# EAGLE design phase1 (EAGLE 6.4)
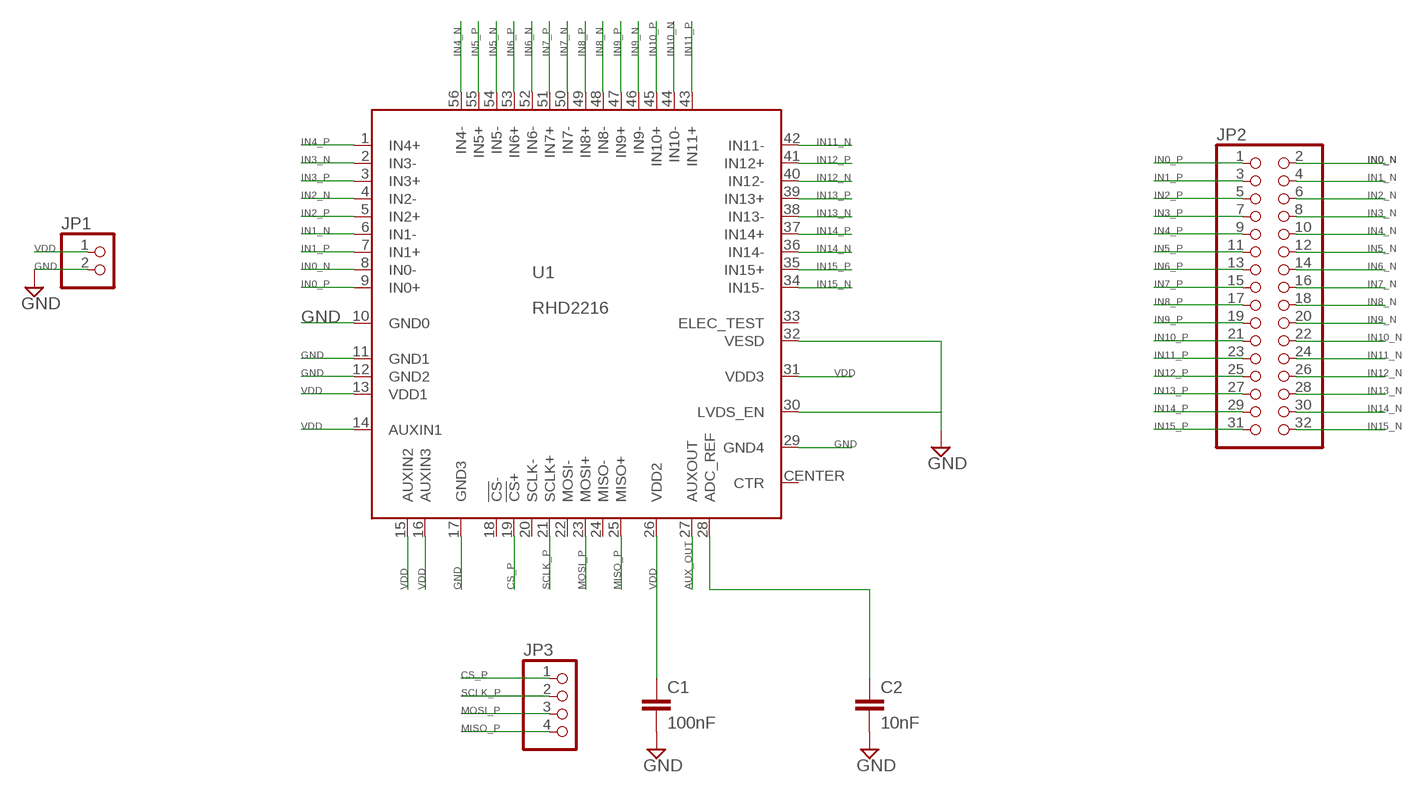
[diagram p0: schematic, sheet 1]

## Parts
C1  100nF  C2.5/2  [C2.5-2]
C2  10nF  C2.5/2  [C2.5-2]
JP1  PINHD-1X2  [1X02]
JP2  PINHD-2X16  [2X16]
JP3  PINHD-1X4  [1X04]
U1  RHD2216  [ZIF_QFN56_8_X_8_MLF00056A1]

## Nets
AUX_OUT: U1.27(AUXOUT)
CS_P: JP3.1 U1.19(!CS!+)
GND: C1.2 C2.2 JP1.2 U1.10(GND0) U1.11(GND1) U1.12(GND2) U1.17(GND3) U1.29(GND4) U1.30(LVDS_EN) U1.32(VESD)
IN0_N: JP2.2 U1.8(IN0-)
IN0_P: JP2.1 U1.9(IN0+)
IN1_N: JP2.4 U1.6(IN1-)
IN1_P: JP2.3 U1.7(IN1+)
IN2_N: JP2.6 U1.4(IN2-)
IN2_P: JP2.5 U1.5(IN2+)
IN3_N: JP2.8 U1.2(IN3-)
IN3_P: JP2.7 U1.3(IN3+)
IN4_N: JP2.10 U1.56(IN4-)
IN4_P: JP2.9 U1.1(IN4+)
IN5_N: JP2.12 U1.54(IN5-)
IN5_P: JP2.11 U1.55(IN5+)
IN6_N: JP2.14 U1.52(IN6-)
IN6_P: JP2.13 U1.53(IN6+)
IN7_N: JP2.16 U1.50(IN7-)
IN7_P: JP2.15 U1.51(IN7+)
IN8_N: JP2.18 U1.48(IN8-)
IN8_P: JP2.17 U1.49(IN8+)
IN9_N: JP2.20 U1.46(IN9-)
IN9_P: JP2.19 U1.47(IN9+)
IN10_N: JP2.22 U1.44(IN10-)
IN10_P: JP2.21 U1.45(IN10+)
IN11_N: JP2.24 U1.42(IN11-)
IN11_P: JP2.23 U1.43(IN11+)
IN12_N: JP2.26 U1.40(IN12-)
IN12_P: JP2.25 U1.41(IN12+)
IN13_N: JP2.28 U1.38(IN13-)
IN13_P: JP2.27 U1.39(IN13+)
IN14_N: JP2.30 U1.36(IN14-)
IN14_P: JP2.29 U1.37(IN14+)
IN15_N: JP2.32 U1.34(IN15-)
IN15_P: JP2.31 U1.35(IN15+)
MISO_P: JP3.4 U1.25(MISO+)
MOSI_P: JP3.3 U1.23(MOSI+)
N$1: C2.1 U1.28(ADC_REF)
SCLK_P: JP3.2 U1.21(SCLK+)
VDD: C1.1 JP1.1 U1.13(VDD1) U1.14(AUXIN1) U1.15(AUXIN2) U1.16(AUXIN3) U1.26(VDD2) U1.31(VDD3)
Unconnected: U1.18(!CS!-) U1.20(SCLK-) U1.22(MOSI-) U1.24(MISO-) U1.33(ELEC_TEST)

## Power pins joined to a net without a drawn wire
CTR: U1.CENTER(CTR)

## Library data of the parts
C1 C2 = capacitor-wima:C: CAPACITOR
JP1 = pinhead:PINHD-1X2: PIN HEADER
JP2 = pinhead:PINHD-2X16: PIN HEADER
JP3 = pinhead:PINHD-1X4: PIN HEADER
U1 = RHD2000:RHD2216

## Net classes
0 default: clearance 0.355 mm

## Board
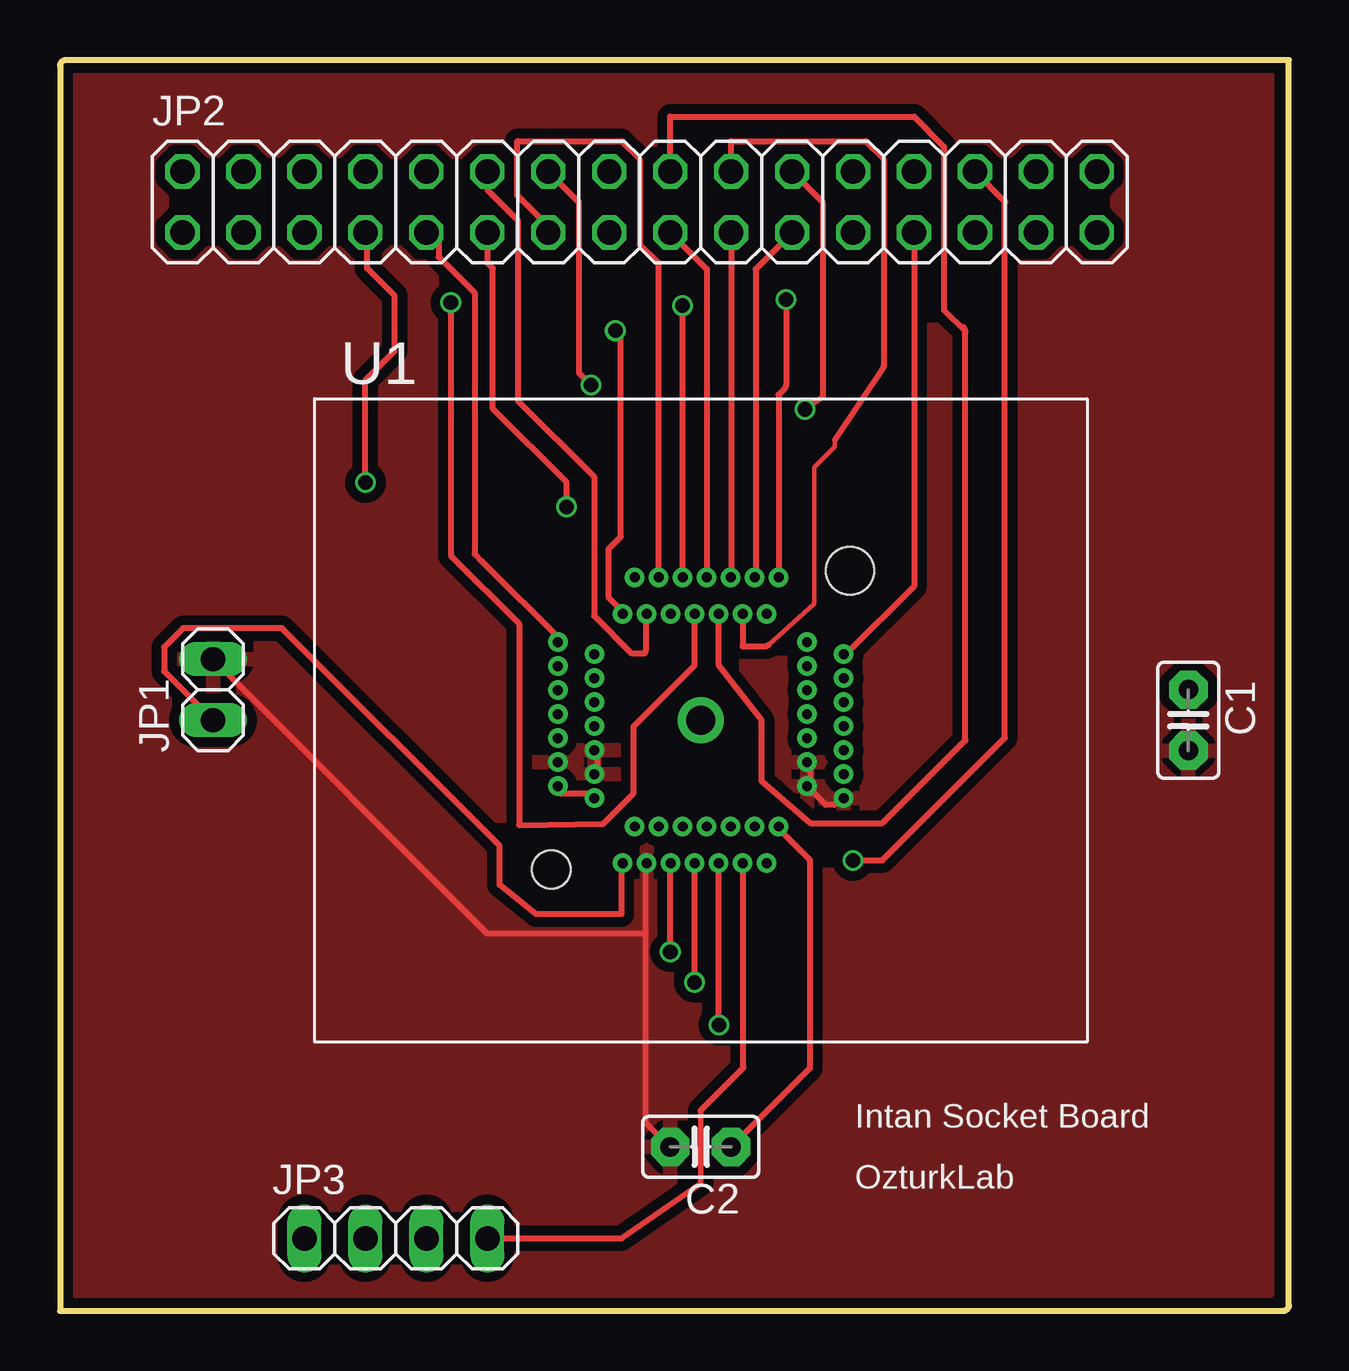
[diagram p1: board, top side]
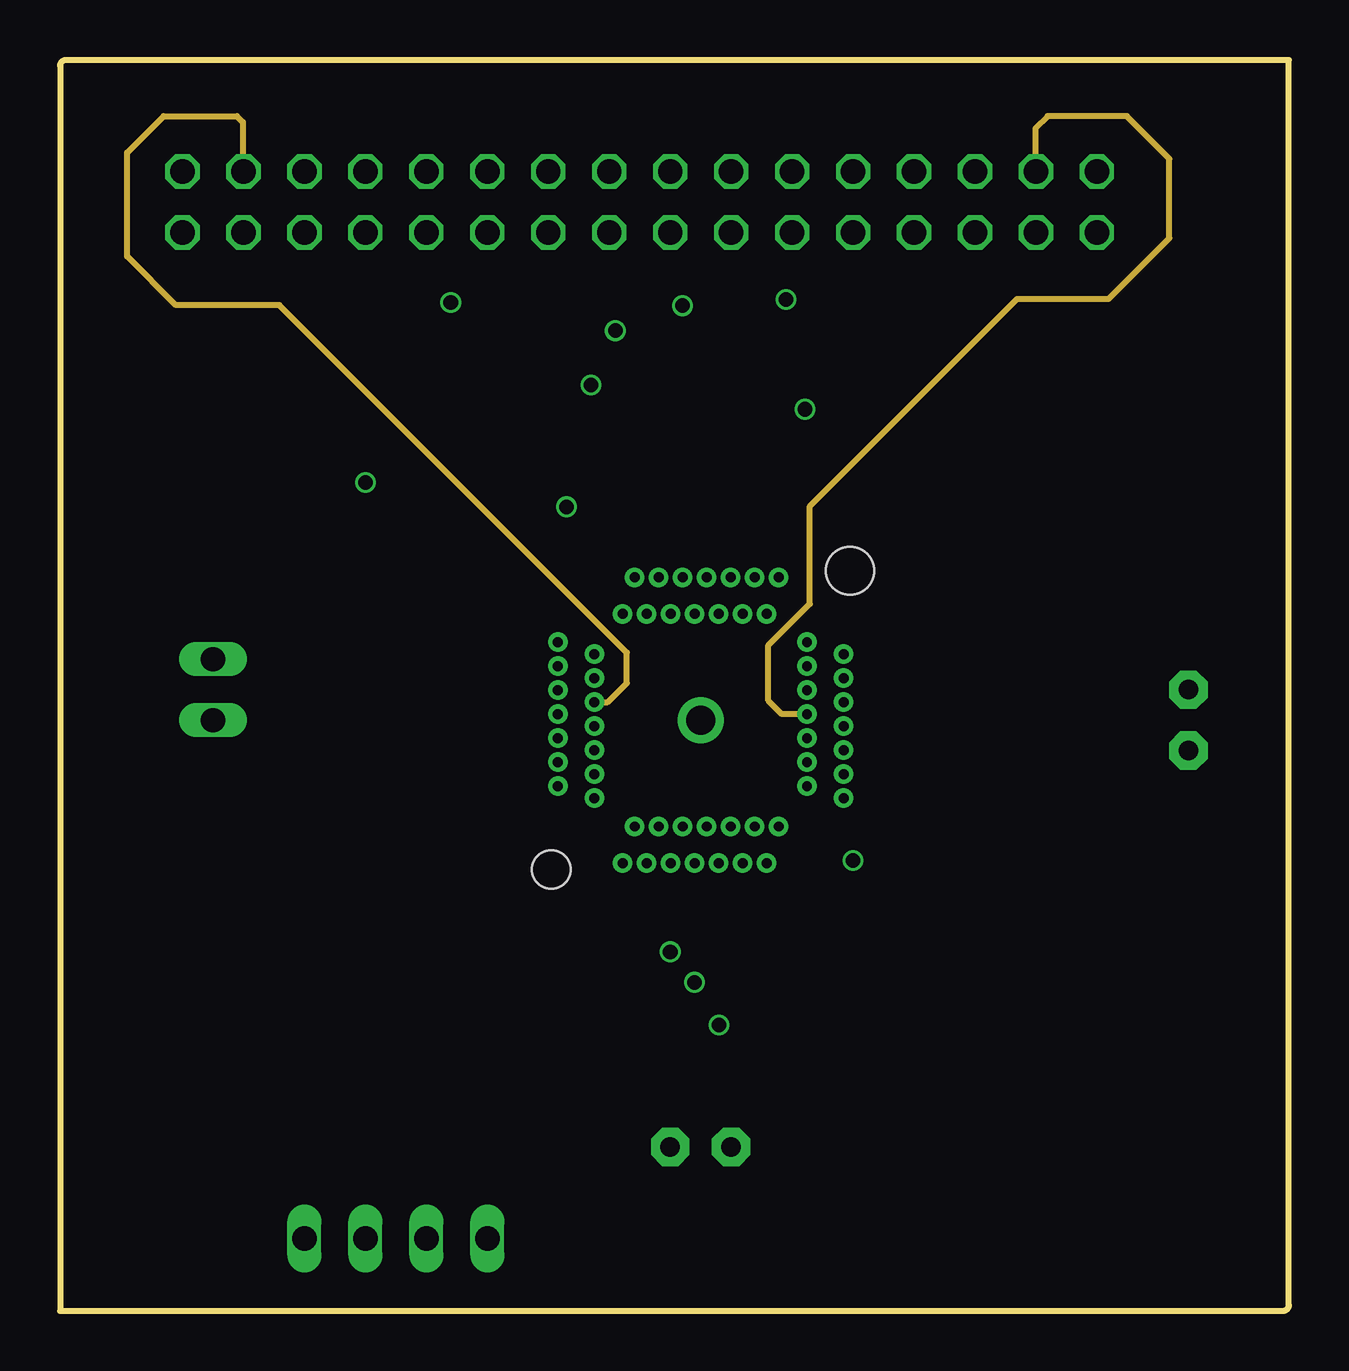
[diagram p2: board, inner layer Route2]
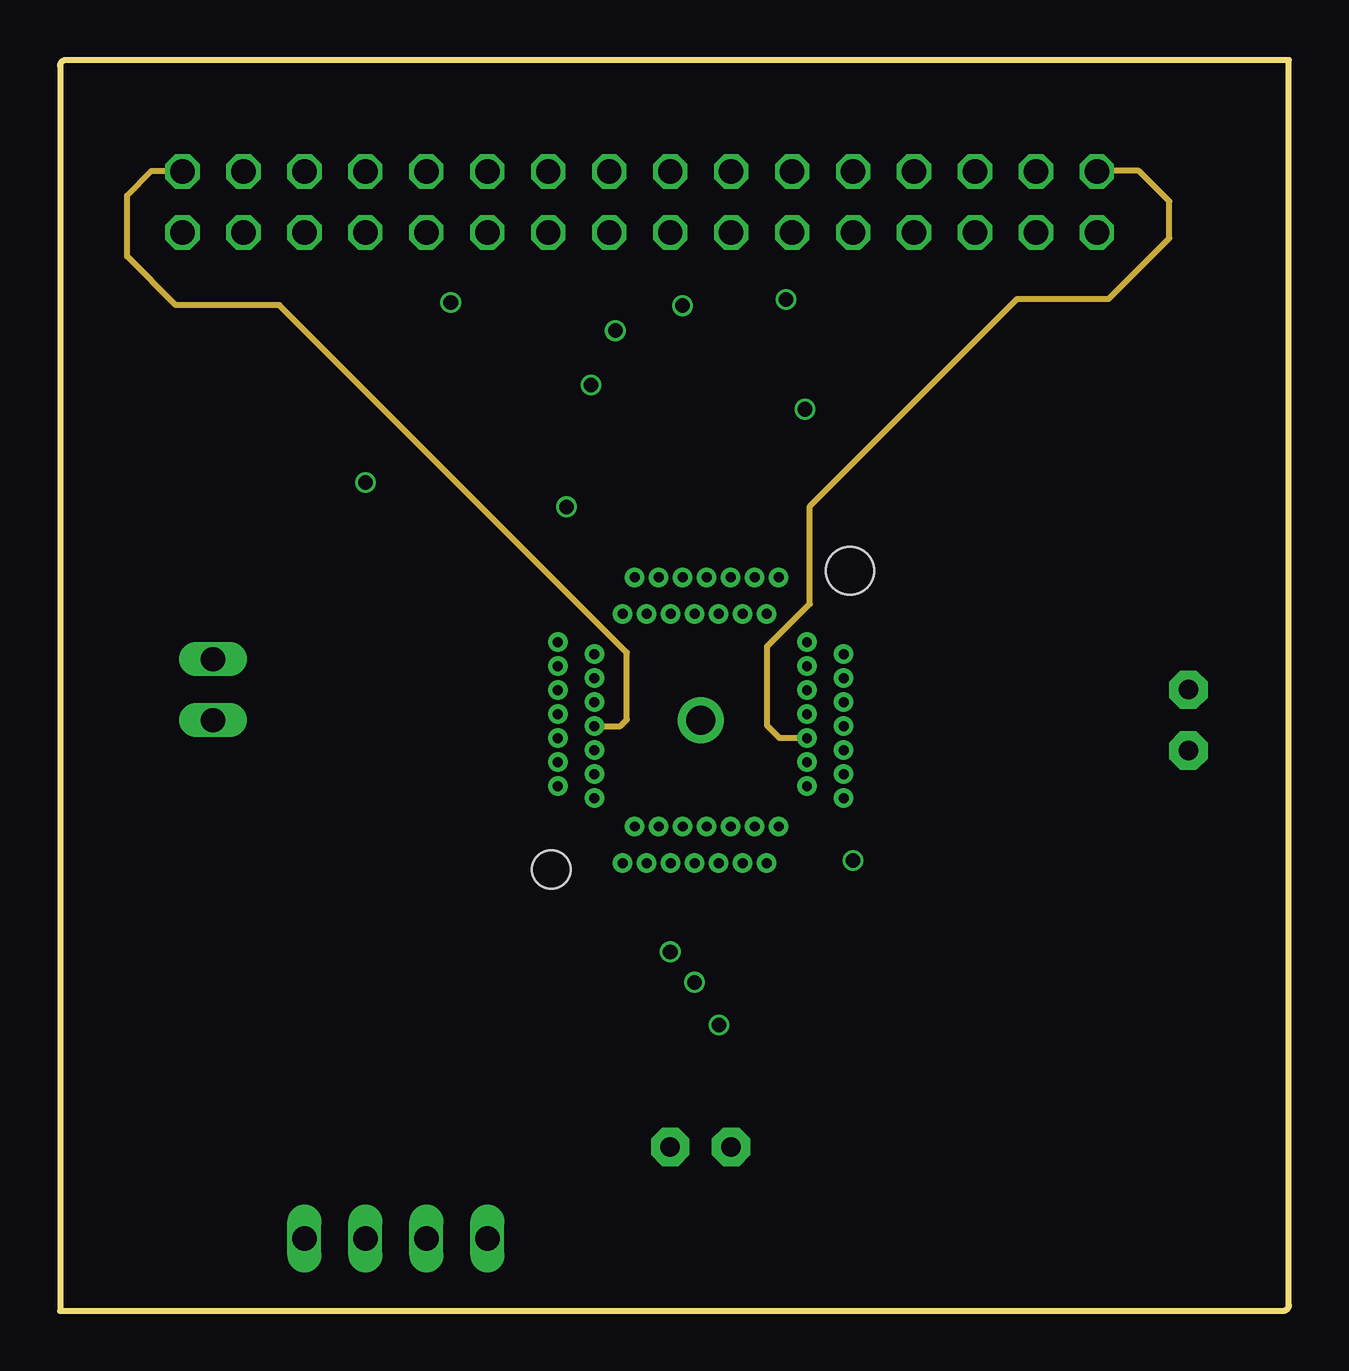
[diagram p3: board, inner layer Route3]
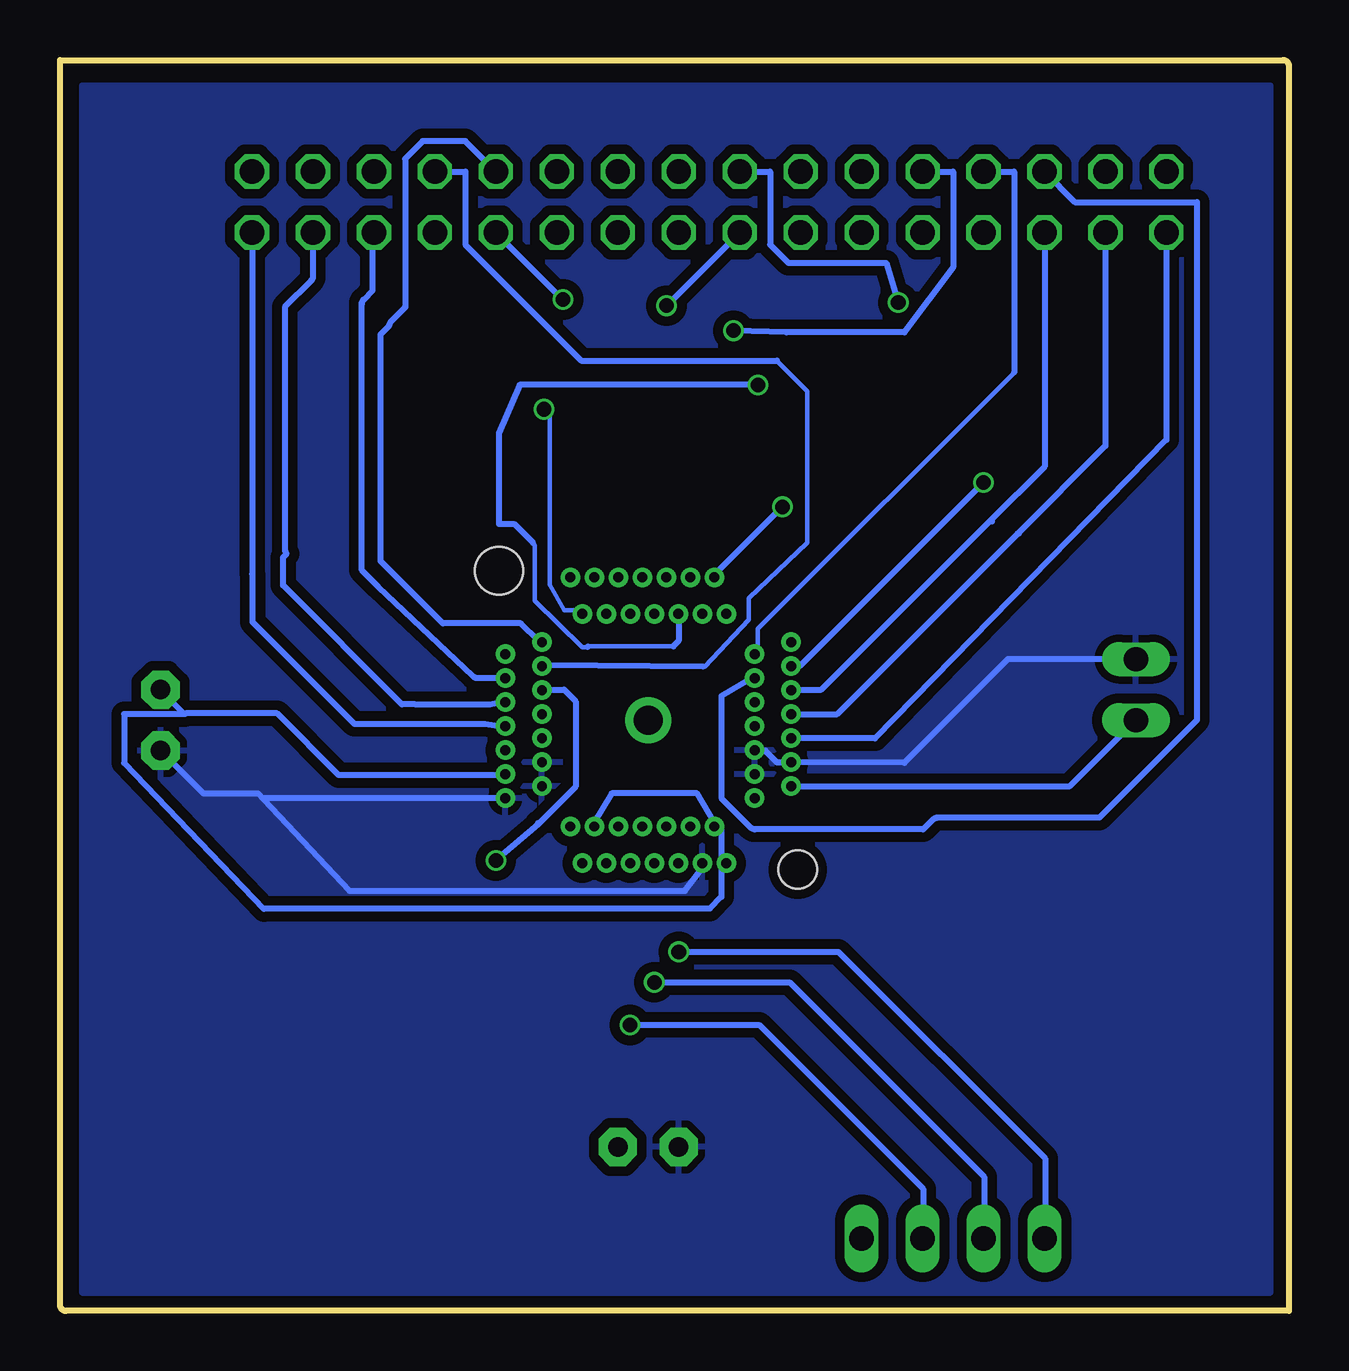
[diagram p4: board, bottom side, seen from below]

Size 51.21 x 52.12 mm. Coordinates in mm from the lower left corner, seen from the top.
Outline: 0,0 50.95,0 arc90 51.21,0.25 51.21,52.12 0.25,52.12 arc90 0,51.87 0,0
Copper layers (1*2*3*16): Top 0.035mm / dielectric 1.5mm / Route2 0.035mm / dielectric 0.15mm / Route3 0.035mm / dielectric 0.2mm / Bottom 0.035mm
Design rules "default *": minimum track width 7mil, minimum drill 6mil, track to track 6mil, track to pad 6mil, pad to pad 6mil, via to via 6mil, smd to smd 5mil, copper to edge 15mil, drill to drill 15mil, minimum pad ring 5mil, minimum via ring 5mil, stop-mask expansion 4mil, vias tented up to drill 0mil, thermal gap 12mil
vRestrict: area 22.4,20.3 to 31.1,28.3

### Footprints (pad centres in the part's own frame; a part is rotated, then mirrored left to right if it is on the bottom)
C2.5-2 = drill 0.813 pad 1.6 octagon: 1 -1.27,0; 2 1.27,0
1X02 = drill 1.016 long: 1 -1.27,0; 2 1.27,0
2X16 = drill 1.016 octagon: 1 -19.05,-1.27; 2 -19.05,1.27; 3 -16.51,-1.27; 4 -16.51,1.27; 5 -13.97,-1.27; 6 -13.97,1.27; 7 -11.43,-1.27; 8 -11.43,1.27; 9 -8.89,-1.27; 10 -8.89,1.27; 11 -6.35,-1.27; 12 -6.35,1.27; 13 -3.81,-1.27; 14 -3.81,1.27; 15 -1.27,-1.27; 16 -1.27,1.27; 17 1.27,-1.27; 18 1.27,1.27; 19 3.81,-1.27; 20 3.81,1.27; 21 6.35,-1.27; 22 6.35,1.27; 23 8.89,-1.27; 24 8.89,1.27; 25 11.43,-1.27; 26 11.43,1.27; 27 13.97,-1.27; 28 13.97,1.27; 29 16.51,-1.27; 30 16.51,1.27; 31 19.05,-1.27; 32 19.05,1.27
1X04 = drill 1.016 long: 1 -3.81,0; 2 -1.27,0; 3 1.27,0; 4 3.81,0
ZIF_QFN56_8_X_8_MLF00056A1 = drill 0.41 pad 0.813: 1 -5.955,3.25; 2 -4.43,2.75; 3 -5.955,2.25; 4 -4.43,1.75; 5 -5.955,1.25; 6 -4.43,0.75; 7 -5.955,0.25; 8 -4.43,-0.25; 9 -5.955,-0.75; 10 -4.43,-1.25; 11 -5.955,-1.75; 12 -4.43,-2.25; 13 -5.955,-2.75; 14 -4.43,-3.25; 15 -3.25,-5.955; 16 -2.75,-4.43; 17 -2.25,-5.955; 18 -1.75,-4.43; 19 -1.25,-5.955; 20 -0.75,-4.43; 21 -0.25,-5.955; 22 0.25,-4.43; 23 0.75,-5.955; 24 1.25,-4.43; 25 1.75,-5.955; 26 2.25,-4.43; 27 2.75,-5.955; 28 3.25,-4.43; 29 5.955,-3.25; 30 4.43,-2.75; 31 5.955,-2.25; 32 4.43,-1.75; 33 5.955,-1.25; 34 4.43,-0.75; 35 5.955,-0.25; 36 4.43,0.25; 37 5.955,0.75; 38 4.43,1.25; 39 5.955,1.75; 40 4.43,2.25; 41 5.955,2.75; 42 4.43,3.25; 43 3.25,5.955; 44 2.75,4.43; 45 2.25,5.955; 46 1.75,4.43; 47 1.25,5.955; 48 0.75,4.43; 49 0.25,5.955; 50 -0.25,4.43; 51 -0.75,5.955; 52 -1.25,4.43; 53 -1.75,5.955; 54 -2.25,4.43; 55 -2.75,5.955; 56 -3.25,4.43 | drill 1.2 pad 1.93: CENTER 0,0 | hole 2: 6.225,6.225 | hole 1.6: -6.225,-6.225

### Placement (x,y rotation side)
C1  47.02,24.61 270 top
C2  26.7,6.83 180 top
JP1  6.38,25.88 90 top
JP2  24.16,46.2 0 top
JP3  14,3.02 0 top
U1  26.7,24.61 0 top

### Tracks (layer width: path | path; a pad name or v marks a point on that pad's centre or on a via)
CS_P  (via drill 0.61)
  Top 0.254: JP3.1 10.19,3.4 | v25.43,14.96 25.43,18.52 U1.19
  Bottom 0.254: v25.43,14.96 18.77,14.96 10.16,6.35 10.16,3.05 JP3.1
GND
  Top 0.254: U1.12 22.38,22.58 22.38,23.34 U1.10 | 24.41,15.72 24.41,7.85 C2.2 | 24.41,15.72 24.41,18.52 U1.17 | U1.30 31.27,22.07 31.27,22.84 U1.32 | 31.27,21.57 31.27,21.82 U1.30 | JP1.2 17.8,15.72 24.41,15.72 | U1.29 32.54,21.36 32.26,21.08 31.91,21.08 U1.30
  Bottom 0.254: 20.85,22.84 U1.11 | U1.10 22.12,23.34 21.82,23.34 21.34,22.86 U1.11 | JP1.2 11.71,27.15 16.03,22.84 U1.11 | C1.2 45.24,21.57 42.95,21.57 42.72,21.31 | 42.72,21.31 39.14,17.5 25.17,17.5 24.41,18.52 U1.17 | U1.29 42.72,21.36 42.72,21.31
  pour Top (isolate 0.406): 0.76,51.44 50.29,51.44 50.29,0.76 0.76,0.76 0.76,51.05
  pour Bottom (isolate 0.406): 1.14,51.05 50.29,51.05 50.29,0.76 0.76,0.76 0.76,51.05
IN0_N
  Route3 0.254: U1.8 23.35,24.36 23.62,24.64 23.62,27.43 9.14,41.91 4.83,41.91 2.79,43.94 2.79,46.48 3.81,47.5 5.08,47.5 JP2.2
IN0_P
  Bottom 0.254: JP2.1 5.11,36.3 17.25,23.85 U1.9
IN1_N
  Route2 0.254: U1.6 22.82,25.36 23.62,26.16 23.62,27.43 9.14,41.91 4.83,41.91 2.79,43.94 2.79,48.26 4.32,49.78 7.37,49.78 7.62,49.53 7.62,47.5 JP2.4
IN1_P
  Bottom 0.254: 11.3,32.38 11.25,32.38 | 11.3,32.38 7.64,36.04 JP2.3 | U1.7 20.6,24.87 18.82,24.87 11.3,32.38
IN2_N
  Bottom 0.254: JP2.6 8.91,46.2 3.83,46.2 3.83,24.61 7.9,20.55 14.65,20.55 arc-45 14.83,20.47 15.24,20.07 22.25,20.07 arc45 22.43,20.14 23.65,21.36 23.65,25.63 22.38,26.39 U1.4
IN2_P
  Bottom 0.254: 12.47,32.89 12.37,32.89 | 12.47,32.89 10.19,35.18 JP2.5 | U1.5 20.6,25.88 19.48,25.88 12.47,32.89
IN3_N
  Bottom 0.178: 22.12,27.41 22.12,28.42 11.46,39.09
  Bottom 0.254: 11.46,39.09 11.46,47.47 JP2.8 | 22.12,27.41 U1.2
IN3_P  (via drill 0.61)
  Top 0.254: v12.72,34.52 12.72,38.79 13.95,40.01 13.95,42.29 12.8,43.43 12.8,44.86 JP2.7
  Bottom 0.254: U1.3 20.6,26.9 20.34,26.9 v12.72,34.52
IN4_N  (via drill 0.61)
  Top 0.254: U1.56 23.39,29.18 22.86,29.72 22.86,31.75 23.37,32.26 23.37,40.62 v23.14,40.84
  Bottom 0.254: v23.14,40.84 20.93,40.77 16.03,40.77 13.99,43.48 13.99,47.47 JP2.10
IN4_P
  Top 0.254: JP2.9 15.77,44.93 15.77,43.92 17.27,42.42 17.27,31.55 17.6,31.22 20.9,27.91 U1.1
IN5_N
  Top 0.254: JP2.12 17.8,46.71 19.07,45.44 19.07,37.92 22.25,34.75 22.25,28.96 23.82,27.38 24.34,27.38 arc45 24.41,27.56 24.41,28.93 U1.54
IN5_P  (via drill 0.61)
  Top 0.254: JP2.11 17.8,43.66 18.03,43.43 18.03,37.59 21.11,34.52 v21.11,33.5
  Bottom 0.254: v21.11,33.5 23.9,30.71 U1.55
IN6_N  (via drill 0.61)
  Top 0.254: v22.12,38.58 21.61,39.09 21.61,46.2 JP2.14
  Bottom 0.178: 25.65,27.69 29.21,27.69 | 31.5,32 31.42,31.88 31.42,29.59 29.44,27.66 29.23,27.66
  Bottom 0.254: U1.52 25.43,28.93 25.43,27.91 25.65,27.69 | v22.12,38.58 32.05,38.58 32.92,36.58 32.92,32.8 32.29,32.8 31.5,32 | 29.21,27.69 29.23,27.66
IN6_P
  Top 0.254: U1.53 24.92,30.71 24.92,43.66 24.16,44.42 24.16,47.98 23.39,48.74 19.07,48.74 19.05,48.72 19.05,46.48 20.34,45.19 JP2.13
IN7_N  (via drill 0.61)
  Top 0.254: v16.28,42.01 16.28,31.47 19.13,28.63 19.13,20.24 22.63,20.3 23.9,21.57 23.9,24.36 26.44,26.9 26.44,28.93 U1.50
  Bottom 0.254: v16.28,42.01 16.79,43.66 20.85,43.66 21.61,44.42 21.61,47.47 JP2.16
IN7_P  (via drill 0.61)
  Top 0.254: v25.93,41.88 25.93,30.71 U1.51
  Bottom 0.254: JP2.15 v25.93,41.88
IN8_N
  Top 0.254: JP2.18 25.43,49.76 35.59,49.76 36.83,48.51 36.83,41.7 37.72,40.81 | U1.48 27.46,28.93 27.46,26.9 29.23,24.61 29.23,22.07 31.27,20.32 34.27,20.32 37.72,23.77 37.72,40.81 | 37.72,40.81 arc45 37.65,40.99
IN8_P
  Top 0.254: JP2.17 26.95,43.41 26.95,30.71 U1.49
IN9_N
  Top 0.178: 29.54,27.76 31.42,29.46 31.42,35.15 32.28,36.01 32.28,36.3
  Top 0.254: 32.28,36.3 34.31,39.34 34.31,47.98 33.55,48.74 27.96,48.74 JP2.20 | U1.46 28.45,27.69 arc45 28.45,27.69 29.36,27.69 arc45 29.54,27.76
IN9_P
  Top 0.254: JP2.19 27.96,30.71 U1.47
IN10_N  (via drill 0.61)
  Top 0.254: v31.04,37.57 31.77,38.08 31.77,46.2 JP2.22
  Bottom 0.178: 29.49,29.18 30.2,29.18 30.81,30.25 30.81,37.8
  Bottom 0.254: 30.76,37.57 v31.04,37.57 30.81,37.8 | 29.49,29.18 U1.44
IN10_P
  Top 0.254: JP2.21 28.98,43.41 28.98,30.71 U1.45
IN11_N
  Bottom 0.254: JP2.24 34.31,48.74 36.09,48.74 36.83,48.01 36.83,41.86 36.8,41.83 37.42,41.22 arc-45 37.49,41.04 37.85,40.69 37.85,31.24 35.26,28.65 32,28.65 31.27,27.91 U1.42
IN11_P  (via drill 0.61)
  Top 0.254: v30.25,42.14 30.25,38.59 arc-45 30.18,38.41 29.95,38.18 U1.43 arc-45 U1.43
  Bottom 0.254: JP2.23 v30.25,42.14
IN12_N
  Bottom 0.178: 24.41,26.85 24.33,26.85 22.5,28.8 22.5,29.69 20.07,32 20.07,38.33 21.34,39.6
  Bottom 0.254: 24.41,26.85 31.01,26.9 U1.40 | 21.34,39.6 29.49,39.6 34.31,44.42 34.31,47.47 JP2.26
IN12_P
  Top 0.254: JP2.25 35.59,30.2 32.79,27.41 U1.41
IN13_N  (via drill 0.61)
  Top 0.254: JP2.28 39.4,46.2 39.37,46.18 39.37,23.88 34.27,18.77 v33.05,18.77
  Bottom 0.254: U1.38 31.01,25.88 30.2,25.88 29.72,25.4 29.72,21.84 31.24,20.32 31.29,20.32 31.27,20.3 v33.05,18.77
IN13_P
  Bottom 0.254: U1.39 33.8,26.36 arc45 33.98,26.44 37.95,30.18 38.63,30.86 38.63,41.96 arc45 38.56,42.14 38.18,42.52 38.18,44.81 arc45 JP2.27
IN14_N
  Route2 0.254: U1.36 30.08,24.86 29.52,25.43 29.52,27.74 31.24,29.46 31.24,33.53 39.88,42.16 43.69,42.16 46.23,44.7 46.23,48.01 44.45,49.78 41.15,49.78 40.64,49.28 40.64,47.5 JP2.30
IN14_P
  Bottom 0.254: U1.37 32.79,25.38 33.3,25.27 36.4,25.27 36.96,25.27 41.91,30.23 41.91,31.4 41.76,31.55 arc45 41.83,31.73 41.83,41.83 40.74,42.93 arc-45 40.66,43.11 JP2.29
IN15_N
  Route3 0.254: U1.34 29.98,23.86 29.46,24.38 29.46,27.69 31.24,29.46 31.24,33.53 39.88,42.16 43.69,42.16 46.23,44.7 46.23,46.23 44.96,47.5 43.23,47.5 JP2.32
IN15_P
  Bottom 0.254: JP2.31 43.2,30.71 43.18,30.68 43.18,28.7 38.94,24.46 33.5,24.46 32.79,24.36 U1.35
MISO_P
  Top 0.229: 26.7,5.31 26.7,8.36
  Top 0.254: 26.7,8.36 28.47,10.13 28.47,18.52 U1.25 | 26.7,5.31 23.39,3.02 JP3.4
MOSI_P  (via drill 0.61)
  Top 0.254: v27.46,11.91 27.46,18.52 U1.23
  Bottom 0.254: v27.46,11.91 22.07,11.91 15.24,5.08 15.24,3.05 JP3.3
N$1
  Top 0.254: C2.1 31.24,10.11 31.24,18.8 30,20.04 U1.28
SCLK_P  (via drill 0.61)
  Top 0.254: v26.44,13.69 26.44,18.52 U1.21
  Bottom 0.254: v26.44,13.69 20.8,13.69 12.7,5.59 12.7,3.05 JP3.2
VDD
  Top 0.254: U1.14 22.12,21.57 20.85,21.57 20.85,21.82 U1.13 | JP1.1 4.34,26.64 4.34,27.66 5.13,28.45 9.25,28.45 18.31,19.38 18.31,17.75 19.84,16.54 23.39,16.54 23.39,18.52 U1.15
  Bottom 0.254: JP1.1 9.12,21.86 U1.13 | U1.26 28.98,20.3 28.22,21.57 24.66,21.57 23.9,20.3 U1.16 23.9,20.04 23.65,20.04 23.65,18.77 U1.15 23.65,18.52 23.65,17.25 24.13,16.76 42.67,16.76 42.7,16.74 48.54,22.84 48.54,24.87 46,24.87 | C1.1 46,24.87 | U1.31 32.79,22.33 39.6,22.33 42.16,24.89 45.97,24.89 46,24.87

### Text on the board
tPlace: Intan Socket Board | OzturkLab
